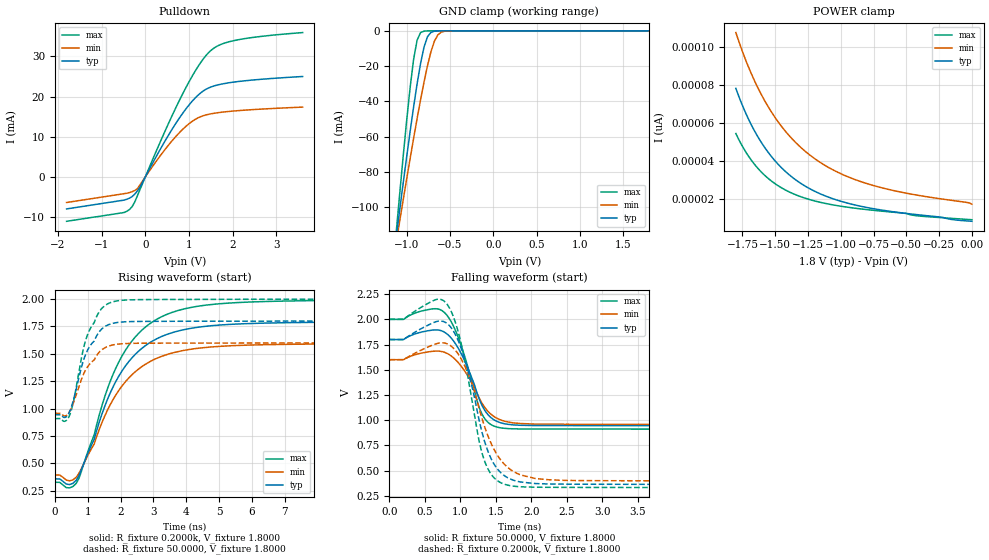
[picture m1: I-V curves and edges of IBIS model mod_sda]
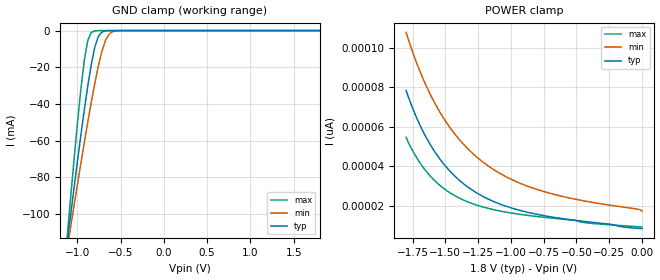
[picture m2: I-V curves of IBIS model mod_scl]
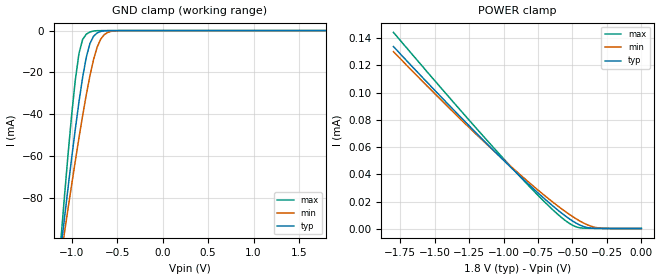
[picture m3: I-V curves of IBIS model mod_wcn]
| IBIS (I/O, Buffer, Information, Specification) Model, officially
| electronic behavioral standard for Buffer structures of digital pins.
[IBIS ver]  4.0
[File name] m24m04e_1d8_tssop8.ibs
[File Rev]  1.0
[Date]   13 Oct 2026
[Source]   CAD & Design Services (Catania) - STMicroelectronics
[Notes]
   (Note1)  This IBIS model includes the TSSOP8 package parasitic data
   (Note2)  This IBIS model has zero Notes and zero Warnings
[Disclaimer]
   Customers are solely responsible for all aspects of their
   own product designs or applications using this IBIS Model.
   STMicroelectronics assumes no liability for Custmer Designs
   and applications associated to this IBIS Model.
   In the use of this IBIS Model Customer shall not modify,
   disassemble, alter this Model in whole or in part.
   If Customers do not accept these terms, the IBIS Model
   may not be used. For any problems or modifications please
   contact STMicroelectronics (www.st.com).
[Copyright] (c) 2026 STMicroelectronics
|   Component M24M04E
[Component] M24M04E
[Manufacturer] STMicroelectronics
[Package]
| variable  typ   min   max
R_pkg   0.0   0.0   0.0
L_pkg   0.0H   0.0H   0.0H
C_pkg   0.0F   0.0F   0.0F
[Pin]  signal_name   model_name   R_pin   L_pin   C_pin
1   NC   NC   0.0   0.0   0.0
2   NC   NC   0.0   0.0   0.0
3   NC   NC   0.0   0.0   0.0
4   VSS   GND   0.0   0.0   0.0
5   SDA   mod_sda   0.0   0.0   0.0
6   SCL   mod_scl   0.0   0.0   0.0
7   WCN   mod_wcn   0.0   0.0   0.0
8   VCC   POWER   0.0   0.0   0.0
[Package Model]  182696_TSSOP8
[Define Package Model]  182696_TSSOP8
[Manufacturer]  STMicroelectronics
[OEM]  STMicroelectronics
[Description]  8 pin TSSOP package
[Number Of Pins]  8
[Pin Numbers]
|Pin Num   Terminal Name
1   | net1
2   | net2
3   | net3
4   | net4_GND
5   | net5
6   | net6
7   | net7
8   | net8_VDD
[Model Data]
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[End Model Data]
[End Package Model]
| Models and submodels in the file (3): mod_sda (I/O_open_drain), mod_scl (Input), mod_wcn (Input)
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|   Model mod_sda
[Model]   mod_sda
Model_type I/O_open_drain
Polarity   Inverting
Enable   Active-High
Vinl   =   0.450V
Vinh   =   1.350V
Vmeas  =   0.900V
Cref   =   30pF
Rref   =   500
Vref   =   1.800V
C_comp   4.636pF   4.427pF   4.855pF
[Temperature Range]   25.0000   85.0000   -40.0000
[Voltage Range]   1.8000V   1.6000V   2.0000V
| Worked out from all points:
|   slope of the pulldown table from 0 to 0.27 V, typ, clamps not added: 49.4 ohm
|   GND clamp passes 1 mA (typ) near -0.72 V on its own axis
|   rising waveform, R_fixture 0.2000k, V_fixture 1.8000: 20-80 % time 1.4ns typ, 1.4ns min, 1.39ns max; typ from 0.36 V to 1.79 V
|   rising waveform, R_fixture 50.0000, V_fixture 1.8000: 20-80 % time 616ps typ, 639ps min, 580ps max; typ from 0.944 V to 1.8 V
|   falling waveform, R_fixture 50.0000, V_fixture 1.8000: 20-80 % time 295ps typ, 314ps min, 274ps max; typ from 1.8 V to 0.944 V
|   falling waveform, R_fixture 0.2000k, V_fixture 1.8000: 20-80 % time 313ps typ, 373ps min, 269ps max; typ from 1.8 V to 0.361 V
[Pulldown]
|Voltage   I(typ)   I(min)   I(max)
-1.8V     -7.942mA   -6.343mA   -11.02mA
-480mV    -5.742mA   -4.143mA   -8.812mA
-300mV    -4.868mA   -3.662mA   -7.363mA
-180mV    -3.46mA    -2.917mA   -4.665mA
420mV     8.349mA    6.387mA    10.62mA
840mV     15.59mA    11.67mA    20.33mA
1.2V      20.27mA    14.66mA    27.34mA
1.38V     21.75mA    15.4mA     30.09mA
1.5V      22.36mA    15.7mA     31.45mA
1.74V     23.09mA    16.09mA    33mA
2.1V      23.7mA     16.47mA    34.06mA
3.6V      24.98mA    17.37mA    35.9mA
[GND_clamp]
|Voltage   I(typ)   I(min)   I(max)
-1.8V     -389.2mA   -332.1mA   -507.3mA
-1.12V    -116.3mA   -119.5mA   -113.3mA
-1.08V    -101mA     -107.4mA   -91.66mA
-1V       -71.13mA   -83.74mA   -50.44mA
-920mV    -42.94mA   -60.76mA   -15.96mA
-880mV    -29.99mA   -49.68mA   -5.261mA
-840mV    -18.43mA   -39.01mA   -1.028mA
-800mV    -9.166mA   -28.93mA   -159.1uA
-760mV    -3.325mA   -19.7mA    -26.96uA
-680mV    -202.6uA   -5.819mA   -1.339uA
-600mV    -10.23uA   -725.2uA   -32.48nA
1.8V      8.512pA    19.96pA    8.401pA
[POWER_clamp]
|Voltage   I(typ)   I(min)   I(max)
-1.8V     78.43pA    107.8pA    54.66pA
-1.74V    67.81pA    96.01pA    46.75pA
-1.68V    58.96pA    85.83pA    40.47pA
-1.62V    51.57pA    77.07pA    35.46pA
-1.54V    43.56pA    67.25pA    30.3pA
-1.46V    37.24pA    59.19pA    26.45pA
-1.38V    32.23pA    52.55pA    23.54pA
-1.2V     24.35pA    41.52pA    19.23pA
-1V       19.06pA    33.56pA    16.45pA
-760mV    15.25pA    27.51pA    14.36pA
-500mV    12.65pA    23.3pA     12.6pA
0V        8.512pA    17.5pA     9.335pA
[Ramp]
| variable   typ   min   max
dV/dt_r   0.5134/0.6085n   0.3853/0.6461n   0.6541/0.5659n
dV/dt_f   0.5133/0.3737n   0.3852/0.3840n   0.6540/0.3349n
R_load = 50.0000
[Rising Waveform]
R_fixture= 0.2000k
V_fixture= 1.8000
V_fixture_min= 1.6000
V_fixture_max= 2.0000
|time   V(typ)   V(min)   V(max)
0s        359.6mV    394.7mV    328.2mV
450ps     307.9mV    341.9mV    277.7mV
650ps     345.9mV    373.4mV    317.6mV
1.2ns     721.3mV    678.5mV    762mV
1.59ns    1.075V     978.3mV    1.171V
1.95ns    1.298V     1.167V     1.427V
2.45ns    1.496V     1.337V     1.654V
3.15ns    1.645V     1.465V     1.823V
5.05ns    1.763V     1.569V     1.958V
10ns      1.792V     1.593V     1.991V
[Rising Waveform]
R_fixture= 50.0000
V_fixture= 1.8000
V_fixture_min= 1.6000
V_fixture_max= 2.0000
|time   V(typ)   V(min)   V(max)
0s        943.9mV    957.6mV    909.6mV
310ps     919.5mV    933.1mV    884.7mV
430ps     958.9mV    962.6mV    925.9mV
550ps     1.06V      1.039V     1.04V
840ps     1.408V     1.29V      1.505V
1ns       1.536V     1.383V     1.677V
1.39ns    1.714V     1.527V     1.9V
1.75ns    1.777V     1.58V      1.973V
2.65ns    1.796V     1.597V     1.995V
10ns      1.799V     1.599V     1.999V
[Falling Waveform]
R_fixture= 50.0000
V_fixture= 1.8000
V_fixture_min= 1.6000
V_fixture_max= 2.0000
|time   V(typ)   V(min)   V(max)
0s        1.8V       1.6V       2V
200ps     1.8V       1.6V       2V
610ps     1.894V     1.683V     2.104V
780ps     1.871V     1.673V     2.064V
980ps     1.702V     1.563V     1.803V
1.3ns     1.154V     1.174V     1.068V
1.41ns    1.039V     1.073V     966.7mV
1.57ns    974mV      1.002V     924mV
2.25ns    946.5mV    960.2mV    912.4mV
10ns      944.3mV    958mV      910mV
[Falling Waveform]
R_fixture= 0.2000k
V_fixture= 1.8000
V_fixture_min= 1.6000
V_fixture_max= 2.0000
|time   V(typ)   V(min)   V(max)
0s        1.8V       1.6V       2V
660ps     1.978V     1.758V     2.197V
820ps     1.955V     1.756V     2.143V
930ps     1.849V     1.693V     1.97V
1.05ns    1.634V     1.556V     1.636V
1.33ns    816mV      960.7mV    618.3mV
1.48ns    558.6mV    702.8mV    425.4mV
1.67ns    428.3mV    530.2mV    355.6mV
2.45ns    365.9mV    403.8mV    333.9mV
10ns      360.8mV    396mV      329.2mV
|   Model mod_scl
[Model]   mod_scl
Model_type Input
Vinl   =   0.450V
Vinh   =   1.350V
C_comp   3.062pF   2.925pF   3.207pF
[Temperature Range]  25.0000   85.0000   -40.0000
[Voltage Range]   1.8000V   1.6000V   2.0000V
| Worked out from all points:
|   GND clamp passes 1 mA (typ) near -0.72 V on its own axis
[GND_clamp]
|Voltage   I(typ)   I(min)   I(max)
-1.8V     -389.2mA   -332.1mA   -507.3mA
-1.12V    -116.3mA   -119.5mA   -113.3mA
-1.08V    -101mA     -107.4mA   -91.66mA
-1V       -71.13mA   -83.74mA   -50.44mA
-920mV    -42.94mA   -60.76mA   -15.96mA
-880mV    -29.99mA   -49.68mA   -5.261mA
-840mV    -18.43mA   -39.01mA   -1.028mA
-800mV    -9.166mA   -28.93mA   -159.1uA
-760mV    -3.325mA   -19.7mA    -26.96uA
-680mV    -202.6uA   -5.819mA   -1.339uA
-600mV    -10.23uA   -725.2uA   -32.48nA
1.8V      8.512pA    19.96pA    8.401pA
[POWER_clamp]
|Voltage   I(typ)   I(min)   I(max)
-1.8V     78.43pA    107.8pA    54.66pA
-1.74V    67.81pA    96.01pA    46.75pA
-1.68V    58.96pA    85.83pA    40.47pA
-1.62V    51.57pA    77.07pA    35.46pA
-1.54V    43.56pA    67.25pA    30.3pA
-1.46V    37.24pA    59.19pA    26.45pA
-1.38V    32.23pA    52.55pA    23.54pA
-1.2V     24.35pA    41.52pA    19.23pA
-1V       19.06pA    33.56pA    16.45pA
-760mV    15.25pA    27.51pA    14.36pA
-500mV    12.65pA    23.3pA     12.6pA
0V        8.512pA    17.5pA     9.335pA
|   Model mod_wcn
[Model]   mod_wcn
Model_type Input
Vinl   =   0.450V
Vinh   =   1.350V
C_comp   3.062pF   2.925pF   3.207pF
[Temperature Range]  25.0000   85.0000   -40.0000
[Voltage Range]   1.8000V   1.6000V   2.0000V
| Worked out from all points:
|   GND clamp passes 1 mA (typ) near -0.71 V on its own axis
[GND_clamp]
|Voltage   I(typ)   I(min)   I(max)
-1.8V     -376.5mA   -320.3mA   -492.8mA
-1.12V    -104.9mA   -108.7mA   -100.7mA
-1.08V    -89.91mA   -96.87mA   -79.55mA
-1V       -60.82mA   -73.61mA   -40.19mA
-960mV    -47.04mA   -62.32mA   -23.49mA
-920mV    -34.1mA    -51.34mA   -10.94mA
-880mV    -22.46mA   -40.79mA   -4.265mA
-800mV    -6.255mA   -21.75mA   -685.8uA
-720mV    -1.127mA   -7.912mA   -49.03uA
-680mV    -409.2uA   -3.995mA   -20.58uA
-560mV    -16.56uA   -306.5uA   -10.48uA
1.8V      349.6nA    257.3nA    493.6nA
[POWER_clamp]
|Voltage   I(typ)   I(min)   I(max)
-1.8V     133.7uA    130uA      144.1uA
-1.42V    93.21uA    91.1uA     99.36uA
-1.08V    58.27uA    58.05uA    60.37uA
-760mV    27.24uA    29.28uA    25.58uA
-640mV    16.56uA    19.39uA    13.7uA
-560mV    10.07uA    13.27uA    6.723uA
-500mV    5.805uA    9.066uA    2.654uA
-460mV    3.444uA    6.529uA    1.073uA
-400mV    1.102uA    3.328uA    447.3nA
-340mV    348.9nA    1.216uA    403.1nA
-260mV    235.3nA    260.1nA    400.7nA
0V        229.6nA    139.2nA    400.6nA
